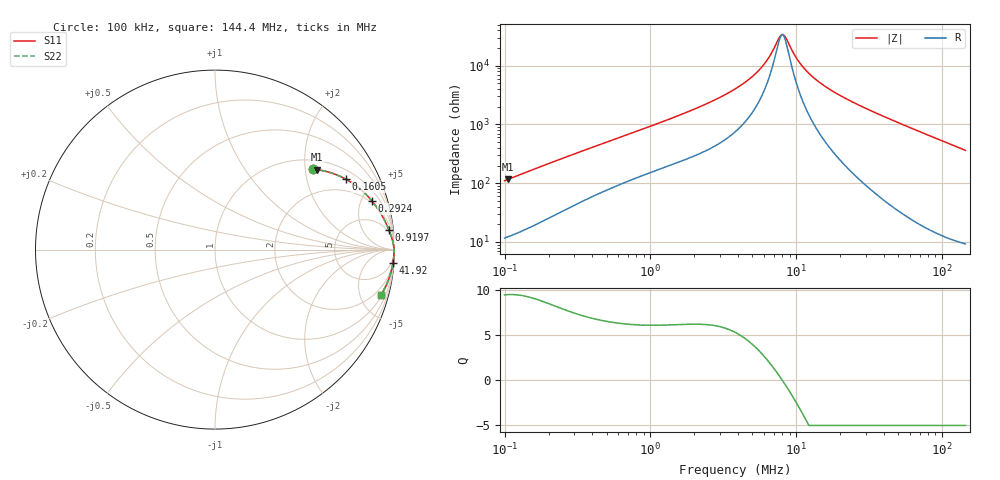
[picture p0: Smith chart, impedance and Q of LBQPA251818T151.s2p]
! LBQPA251818T151  S-PARAMETER MODEL  ( General Type )
! Model Generated by TAIYO YUDEN Corporation (http://www.ty-top.com)
! Version 1.0
! TAIYO YUDEN Control No. 191025NI43SB-FBB
! Copyright(c) 2019 TAIYO YUDEN CO.,LTD. All Rights Reserved.
! Product Description (link to TY-COMPAS)
! https://ds.yuden.co.jp/TYCOMPAS/or/detail?pn=LBQPA251818T151K&u=M
! Products Name : Inductors
! Characteristics :
!  Inductance : 150 uH , SRF(min) : 7.0 MHz , DC Resistance(max) : 7.93 Ohm
!  Rated Current : Saturation :140 mA , Temp Rise : 95 mA (20 degC)
!  Case Size : 2.5 x 1.8 / 0.098 x 0.071 [mm/inch] , Thickness : 1.8 / 0.071 [mm/inch]
!  (Conditions: Temperature = 25 degC , DC Bias Current/Voltage = 0A / 0V)
! External Node Assignments :
!  1  o---GGG---o  2
! GND o---------o GND
! Frequency Range : 0.1MHz  -  144.390904MHz  [ 402 STEP ]
# MHz S RI R 50
! Freq[MHz].  S11 Real  S11 Imag  S21 Real  S21 Imag  S12 Real  S12 Imag  S22 Real  S22 Imag
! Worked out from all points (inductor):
!   401 points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, 100 kHz to 144.4 MHz, reference 50 ohm
!   read as one part in series: L = 174 uH near 103.7 kHz
!   highest Q = 9.45 at 105.6 kHz (marker M1), where L = 175 uH
!   self-resonance near 8.01 MHz
!   S11 on the Smith chart (normalised r, x): 100 kHz: 1.23, +2.20; 160.5 kHz: 1.39, +3.47; 292.4 kHz: 1.81, +6.08; 919.7 kHz: 4, +17; 41.92 MHz: 2, -26; 144.4 MHz: 1.19, -7.25
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0.1  0.5447 0.4478  0.4553 -0.4478  0.4553 -0.4478  0.5447 0.4478
0.105608  0.5685 0.4452  0.4315 -0.4452  0.4315 -0.4452  0.5685 0.4452
0.160461  0.7311 0.3914  0.2689 -0.3914  0.2689 -0.3914  0.7311 0.3914
0.292437  0.8747 0.2708  0.1253 -0.2708  0.1253 -0.2708  0.8747 0.2708
0.338238  0.8959 0.2434  0.1041 -0.2434  0.1041 -0.2434  0.8959 0.2434
0.919729  0.9694 0.1087  0.0306 -0.1087  0.0306 -0.1087  0.9694 0.1087
1.144052  0.9766 0.0899  0.0234 -0.0899  0.0234 -0.0899  0.9766 0.0899
2.368099  0.9907 0.0444  0.00926 -0.0444  0.00926 -0.0444  0.9907 0.0444
3.869624  0.9949 0.0236  0.0051 -0.0236  0.0051 -0.0236  0.9949 0.0236
4.813433  0.9959 0.016  0.00409 -0.016  0.00409 -0.016  0.9959 0.016
5.773557  0.9965 0.0101  0.00352 -0.0101  0.00352 -0.0101  0.9965 0.0101
6.557456  0.9968 0.00612  0.00323 -0.00612  0.00323 -0.00612  0.9968 0.00612
7.584487  0.997 0.00168  0.003 -0.00168  0.003 -0.00168  0.997 0.00168
8.00982  0.9971 2.86e-05  0.00294 -2.86e-05  0.00294 -2.86e-05  0.9971 2.86e-05
8.459005  0.9971 -0.00163  0.00288 0.00163  0.00288 0.00163  0.9971 -0.00163
9.607519  0.9972 -0.00553  0.00281 0.00553  0.00281 0.00553  0.9972 -0.00553
10.52217  0.9972 -0.00838  0.00279 0.00838  0.00279 0.00838  0.9972 -0.00838
12.85266  0.9972 -0.0149  0.00284 0.0149  0.00284 0.0149  0.9972 -0.0149
19.88681  0.9964 -0.0317  0.00355 0.0317  0.00355 0.0317  0.9964 -0.0317
41.91969  0.9913 -0.0764  0.00867 0.0764  0.00867 0.0764  0.9913 -0.0764
43.47261  0.9908 -0.0794  0.00917 0.0794  0.00917 0.0794  0.9908 -0.0794
144.3909  0.9238 -0.2528  0.0762 0.2528  0.0762 0.2528  0.9238 -0.2528
